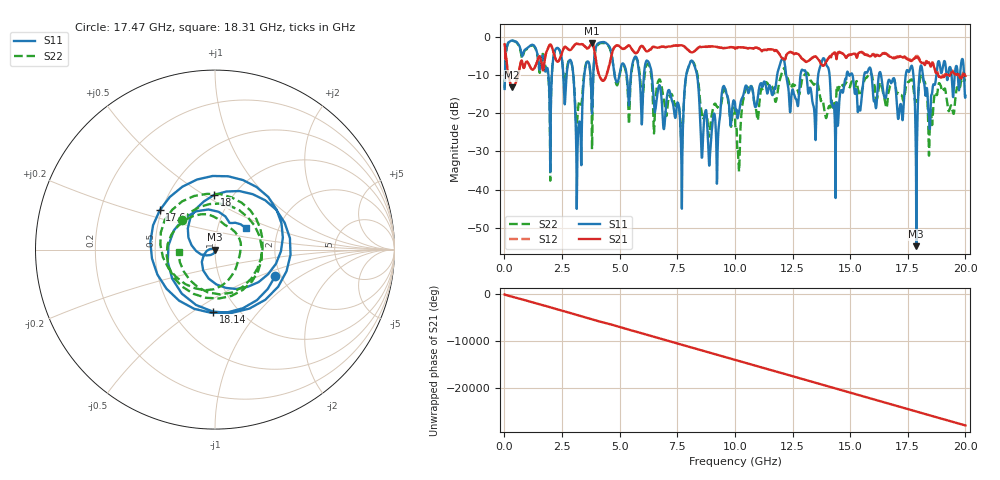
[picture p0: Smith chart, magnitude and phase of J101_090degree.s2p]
!Keysight Technologies,N5222A,MY51421036,A.10.65.16
!Date: Friday, March 31, 2023 14:49:54
!Correction: S11(Full 2 Port(1,2))
!S21(Full 2 Port(1,2))
!S12(Full 2 Port(1,2))
!S22(Full 2 Port(1,2))
!S2P File: Measurements: S11, S21, S12, S22:
# Hz S  dB  R 50
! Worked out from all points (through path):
!   2000 points, 10 MHz to 20 GHz, reference 50 ohm
!   highest |S21| = -1.60 dB at 3.8 GHz (marker M1); lowest = -13.2 dB at 340 MHz (marker M2)
!   group delay of S21, straight-line fit = 3.9 ns
!   lowest |S11| = -54.8 dB at 17.87 GHz (marker M3), VSWR 1.00, Z = 49.8 + j0.0231 ohm
!   |S11| at or under -10 dB: 6.395 GHz to 7.89 GHz (1.495 GHz wide, 20.9 % of centre); 8.359 GHz to 11.83 GHz (3.474 GHz wide, 34.4 % of centre); 16.34 GHz to 17.41 GHz (1.072 GHz wide, 6.35 % of centre)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
!   |S22| runs from -37.7 to -1.0 dB; largest |S21 - S12| = 0.023
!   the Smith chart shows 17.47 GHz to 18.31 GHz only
!   S11 on the Smith chart (normalised r, x): 17.47 GHz: 1.87, -0.64; 17.6 GHz: 0.49, +0.25; 18 GHz: 0.82, +0.55; 18.14 GHz: 0.77, -0.61; 18.31 GHz: 1.36, +0.34
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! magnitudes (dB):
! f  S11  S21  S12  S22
! 10 MHz  -13.6  -1.9  -1.9  -13.5
! 340 MHz  -1.0  -13.2  -13.2  -1.0
! 1.96 GHz  -16.5  -2.1  -2.1  -17.8
! 2.86 GHz  -6.0  -3.4  -3.4  -6.2
! 3.15 GHz  -39.9  -1.8  -1.8  -23.2
! 3.35 GHz  -28.5  -1.9  -1.8  -17.5
! 3.8 GHz  -20.1  -1.6  -1.5  -29.4
! 4.23 GHz  -1.4  -11.4  -11.3  -1.6
! 6.68 GHz  -13.3  -2.8  -2.7  -11.5
! 7.68 GHz  -33.1  -2.2  -2.2  -28.9
! 8.17 GHz  -6.5  -4.0  -4.0  -6.4
! 8.91 GHz  -31.8  -2.5  -2.5  -24.9
! 10.01 GHz  -17.7  -3.1  -3.0  -21.8
! 13.34 GHz  -15.8  -5.6  -5.5  -11.8
! 16.67 GHz  -11.3  -5.0  -4.9  -14.3
! 17.47 GHz  -8.7  -5.8  -5.7  -12.2
! 17.6 GHz  -8.4  -6.2  -6.0  -11.3
! 17.87 GHz  -54.8  -5.3  -5.0  -16.6
! 18 GHz  -10.3  -6.0  -5.7  -12.3
! 18.14 GHz  -9.2  -6.9  -6.6  -10.4
! 18.31 GHz  -13.6  -6.5  -6.3  -13.9
! 20 GHz  -15.4  -10.2  -9.8  -10.9
